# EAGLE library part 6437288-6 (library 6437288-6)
Header vert 26 way 4 row Tab Superseal Source: Datasheet
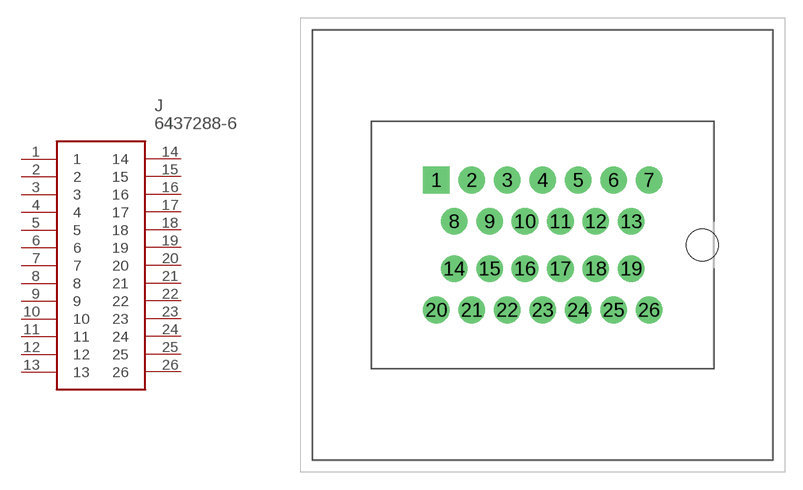
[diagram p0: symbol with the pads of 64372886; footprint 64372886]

Designator prefix J

## 6437288-6 (Description: Header vert 26 way 4 row Tab Superseal; Height: 24.7mm; Manufacturer_Name: TE Connectivity; Manufacturer_Part_Number: 6437288-6; Mouser_Part_Number: 571-6437288-6; Mouser_Price-Stock: https://www.mouser.co.uk/ProductDetail/TE-Connectivity-AMP/6437288-6?qs=PZo9TgaVsd8aPKRekLZQ8g%3D%3D)  [64372886]
1  1
2  2
3  3
4  4
5  5
6  6
7  7
8  8
9  9
10  10
11  11
12  12
13  13
14  14
15  15
16  16
17  17
18  18
19  19
20  20
21  21
22  22
23  23
24  24
25  25
26  26

## Footprint 64372886 (pad centres in mm)
6437288-6-2
drill 1.5 pad 2.25 square: 1 0,0
drill 1.5 pad 2.25: 2 3,0; 3 6,0; 4 9,0; 5 12,0; 6 15,0; 7 18,0; 8 1.5,-3.5; 9 4.5,-3.5; 10 7.5,-3.5; 11 10.5,-3.5; 12 13.5,-3.5; 13 16.5,-3.5; 14 1.5,-7.5; 15 4.5,-7.5; 16 7.5,-7.5; 17 10.5,-7.5; 18 13.5,-7.5; 19 16.5,-7.5; 20 0,-11; 21 3,-11; 22 6,-11; 23 9,-11; 24 12,-11; 25 15,-11; 26 18,-11
hole 2.7 at 22.5,-5.5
